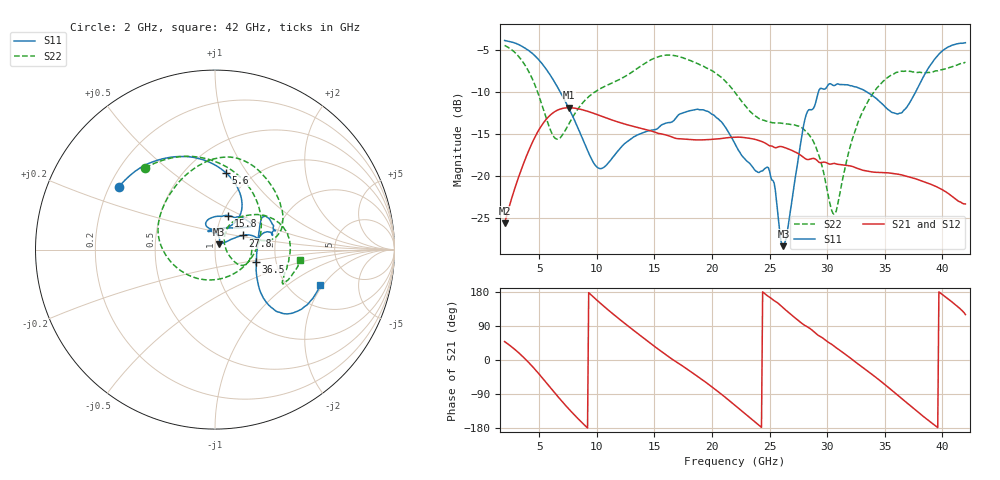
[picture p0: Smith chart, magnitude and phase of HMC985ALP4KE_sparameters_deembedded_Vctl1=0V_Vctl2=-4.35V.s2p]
!s2p File: Measurements: S11, S21, S12, S22
# GHz S dB R 50.0
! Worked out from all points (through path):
!   401 points, 2 GHz to 42 GHz, reference 50 ohm
!   highest |S21| = -11.89 dB at 7.6 GHz (marker M1); lowest = -25.7 dB at 2 GHz (marker M2)
!   lowest |S11| = -28.4 dB at 26.2 GHz (marker M3), VSWR 1.08, Z = 52.3 + j3.17 ohm
!   |S11| at or under -10 dB: 6.821 GHz to 29.25 GHz (22.43 GHz wide, 124 % of centre); 33.42 GHz to 37.69 GHz (4.271 GHz wide, 12 % of centre)
!   |S22| runs from -24.6 to -4.5 dB; largest |S21 - S12| = 0.00021
!   S11 on the Smith chart (normalised r, x): 2 GHz: 0.24, +0.28; 5.6 GHz: 0.76, +0.80; 15.8 GHz: 1.07, +0.42; 27.8 GHz: 1.34, +0.22; 36.5 GHz: 1.57, -0.23; 42 GHz: 2.94, -1.89
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2  -3.88 147.0  -25.66 48.6  -25.67 48.6  -4.47 130.5
3.6  -4.66 120.3  -18.70 8.4  -18.70 8.4  -6.48 84.9
4.7  -5.80 99.5  -15.21 -26.8  -15.22 -26.8  -9.42 43.3
5.6  -7.29 81.9  -13.29 -59.1  -13.30 -59.1  -13.06 -3.8
6.5  -9.22 66.5  -12.24 -92.0  -12.25 -92.0  -15.62 -69.1
7.6  -12.03 54.8  -11.89 -130.1  -11.90 -130.2  -13.76 -135.9
8.7  -15.38 55.0  -12.12 -164.8  -12.12 -164.8  -11.44 -170.3
10.4  -19.13 89.6  -12.90 147.4  -12.90 147.4  -9.55 162.4
15.4  -14.22 75.7  -14.97 27.4  -14.97 27.4  -5.79 87.0
15.8  -13.83 68.7  -15.06 18.5  -15.07 18.5  -5.66 81.9
19.4  -12.23 33.3  -15.71 -57.4  -15.72 -57.4  -7.06 34.9
22  -16.19 51.1  -15.40 -119.7  -15.40 -119.7  -10.08 9.9
24.9  -19.04 104.7  -16.35 167.6  -16.35 167.6  -13.56 13.2
26.2  -28.38 52.7  -16.59 137.2  -16.59 137.2  -13.78 -2.6
27.8  -15.23 27.2  -17.65 96.8  -17.65 96.7  -14.28 -24.7
28.7  -12.11 12.6  -17.94 78.6  -17.94 78.6  -15.64 -31.6
30.6  -9.26 19.5  -18.52 36.7  -18.53 36.7  -24.57 16.1
32.8  -9.59 33.9  -19.20 -13.3  -19.20 -13.3  -13.21 53.2
35.4  -12.22 11.7  -19.67 -74.5  -19.67 -74.5  -8.16 21.2
36.5  -12.47 -16.7  -19.91 -102.4  -19.91 -102.4  -7.55 7.1
39.5  -5.85 -43.7  -21.31 -175.9  -21.32 -176.0  -7.50 -26.3
42  -4.16 -18.6  -23.36 119.9  -23.36 119.8  -6.46 -7.1
